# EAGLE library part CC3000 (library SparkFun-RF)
Texas Instruments CC3000 WiFi Module The CC3000 from TI (Texas Instruments) is a self-contained wireless network processor that makes incorporating internet connectivity into your project simple. Instead of the more standard UART communication method, the CC3000 module utilizes an SPI interface allowing you, the user, to control the flow of data as you please. SparkFun Products WiFi SMD Module - CC3000 (WRL-12820) SparkFun WiFi Breakout - CC3000 (WRL-12072) SparkFun WiFi Shield - CC3000 (WRL-12071)
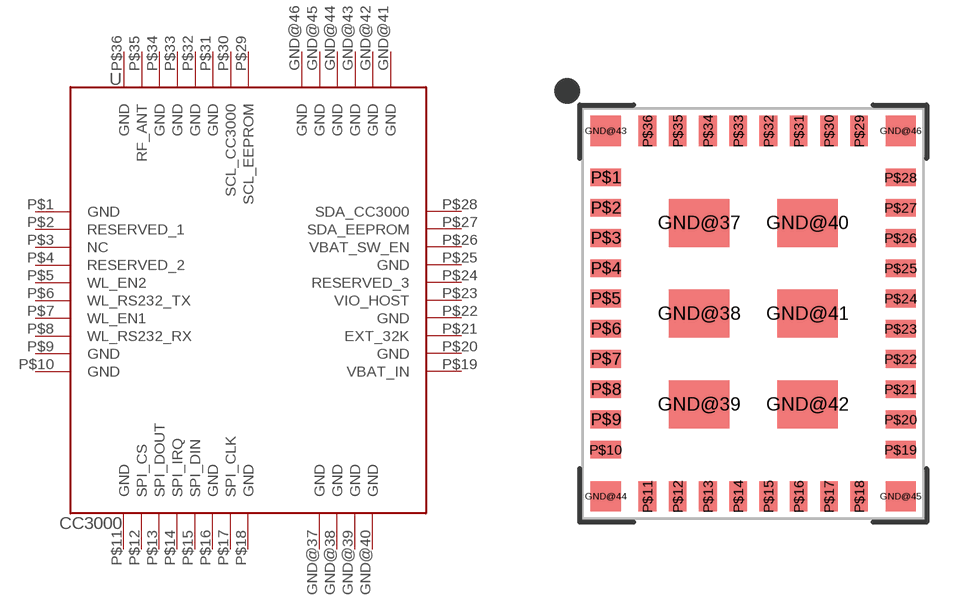
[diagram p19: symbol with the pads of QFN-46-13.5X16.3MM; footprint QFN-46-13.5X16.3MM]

Designator prefix -

## CC3000 (PROD_ID: IC-12643; SF_ID: WRL-13444)  [QFN-46-13.5X16.3MM]
GND@37  GND
GND@38  GND
GND@39  GND
GND@40  GND
GND@41  GND
GND@42  GND
GND@43  GND
GND@44  GND
GND@45  GND
GND@46  GND
P$1  GND
P$2  RESERVED_1
P$3  NC
P$4  RESERVED_2
P$5  WL_EN2
P$6  WL_RS232_TX
P$7  WL_EN1
P$8  WL_RS232_RX
P$9  GND
P$10  GND
P$11  GND
P$12  SPI_CS
P$13  SPI_DOUT
P$14  SPI_IRQ
P$15  SPI_DIN
P$16  GND
P$17  SPI_CLK
P$18  GND
P$19  VBAT_IN
P$20  GND
P$21  EXT_32K
P$22  GND
P$23  VIO_HOST
P$24  RESERVED_3
P$25  GND
P$26  VBAT_SW_EN
P$27  SDA_EEPROM
P$28  SDA_CC3000
P$29  SCL_EEPROM
P$30  SCL_CC3000
P$31  GND
P$32  GND
P$33  GND
P$34  GND
P$35  RF_ANT
P$36  GND

## Footprint QFN-46-13.5X16.3MM (pad centres in mm)
Texas Instruments CC3000 Wi-Fi Module Size: 16.3 x 13.5 x 2.0 mm Datasheet
smd 2.4 x 1.9: GND@37 -2.15,3.6; GND@38 -2.15,0; GND@39 -2.15,-3.6; GND@40 2.15,3.6; GND@41 2.15,0; GND@42 2.15,-3.6
smd 1.2 x 1.2: GND@43 -5.85,7.25; GND@44 -5.85,-7.25; GND@45 5.85,-7.25; GND@46 5.85,7.25
smd 1.2 x 0.7: P$1 -5.85,5.4; P$2 -5.85,4.2; P$3 -5.85,3; P$4 -5.85,1.8; P$5 -5.85,0.6; P$6 -5.85,-0.6; P$7 -5.85,-1.8; P$8 -5.85,-3; P$9 -5.85,-4.2; P$10 -5.85,-5.4; P$19 5.85,-5.4; P$20 5.85,-4.2; P$21 5.85,-3; P$22 5.85,-1.8; P$23 5.85,-0.6; P$24 5.85,0.6; P$25 5.85,1.8; P$26 5.85,3; P$27 5.85,4.2; P$28 5.85,5.4
smd 0.7 x 1.2: P$11 -4.2,-7.25; P$12 -3,-7.25; P$13 -1.8,-7.25; P$14 -0.6,-7.25; P$15 0.6,-7.25; P$16 1.8,-7.25; P$17 3,-7.25; P$18 4.2,-7.25; P$29 4.2,7.25; P$30 3,7.25; P$31 1.8,7.25; P$32 0.6,7.25; P$33 -0.6,7.25; P$34 -1.8,7.25; P$35 -3,7.25; P$36 -4.2,7.25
